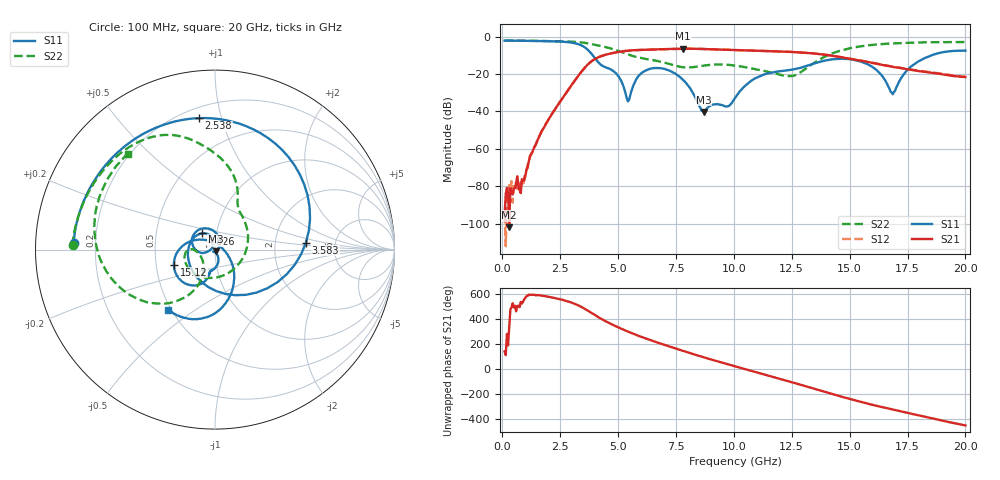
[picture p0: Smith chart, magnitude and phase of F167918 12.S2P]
!  2-Port S-parameters saved by WinCal
! VAR MeasName=S-Parameters (CALIBRATED_DATA) read from VNA (N5242A)
! VAR MeasDate=2016-11-22 10:25:23
! VAR NAME=F167918 12
! VAR FILENAME=F167918 12.S2P
! VAR DATE=2016-11-22 10:25:23
! VAR PHYS_PORTS=1,2
# Hz S DB R 50
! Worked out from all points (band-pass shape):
!   401 points, 100 MHz to 20 GHz, reference 50 ohm
!   highest |S21| = -6.40 dB at 7.811 GHz (marker M1); lowest = -102.0 dB at 299 MHz (marker M2)
!   |S21| within 3 dB of the highest: 4.538 GHz to 13.77 GHz (9.229 GHz wide, 101 % of centre)
!   lowest |S11| = -40.2 dB at 8.707 GHz (marker M3), VSWR 1.02, Z = 50.4 - j0.895 ohm
!   |S11| at or under -10 dB: 3.91 GHz to 18.53 GHz (14.62 GHz wide, 130 % of centre)
!   |S22| runs from -21.1 to -2.0 dB; largest |S21 - S12| = 0.0033
!   S11 on the Smith chart (normalised r, x): 100 MHz: 0.12, +0.02; 2.538 GHz: 0.26, +0.85; 3.583 GHz: 3.03, +0.32; 4.826 GHz: 0.85, +0.16; 15.12 GHz: 0.62, -0.11; 20 GHz: 0.48, -0.39
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1e8  -2.07 177.3  -95.21 140.4  -95.16 15.5  -2.00 178.3
2.99e8  -2.09 172.0  -101.95 -30.9  -79.55 117.6  -2.03 175.0
8.4625e8  -2.18 157.3  -76.30 165.3  -77.27 170.1  -2.12 166.2
1.5925e9  -2.31 135.3  -53.51 -127.6  -53.36 -130.8  -2.24 154.1
2.53775e9  -2.64 97.0  -34.04 -162.5  -33.99 -163.3  -2.44 136.7
3.43325e9  -4.76 24.4  -18.49 135.7  -18.51 135.7  -3.07 114.8
3.5825e9  -5.88 4.4  -16.30 120.1  -16.31 120.2  -3.32 110.6
3.9805e9  -11.12 -66.1  -12.09 74.0  -12.05 74.0  -4.28 100.2
4.82625e9  -18.67 129.3  -8.59 -11.2  -8.58 -11.5  -6.80 79.6
5.42325e9  -34.63 141.7  -7.49 -60.7  -7.49 -60.8  -9.44 68.0
5.9705e9  -19.87 -176.2  -7.07 -101.0  -7.08 -101.3  -11.34 61.5
6.7665e9  -16.76 135.7  -6.74 -152.9  -6.75 -153.1  -13.18 37.7
7.81125e9  -23.13 71.2  -6.40 143.9  -6.43 144.0  -16.36 -39.1
8.70675e9  -40.23 -65.7  -6.58 92.3  -6.59 92.2  -15.46 -115.6
1.005e10  -32.81 -71.4  -7.13 20.4  -7.14 20.5  -15.47 -171.6
1.1841e10  -18.73 -98.3  -7.84 -72.7  -7.81 -72.3  -19.76 -173.7
1.338325e10  -14.71 -107.5  -8.88 -155.6  -8.84 -155.4  -14.68 -114.9
1.51245e10  -12.27 -159.9  -12.03 112.5  -11.99 112.4  -5.89 -146.9
1.606975e10  -16.89 160.8  -14.20 67.1  -14.26 67.5  -4.27 -167.5
1.67165e10  -27.71 101.9  -15.71 38.6  -15.75 39.3  -3.67 -179.9
1.815925e10  -11.93 -68.5  -18.66 -21.1  -18.50 -20.6  -3.03 156.7
2e10  -7.42 -128.0  -21.61 -94.9  -21.42 -95.2  -2.84 132.2
